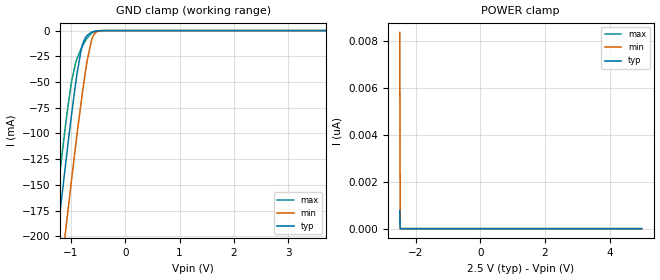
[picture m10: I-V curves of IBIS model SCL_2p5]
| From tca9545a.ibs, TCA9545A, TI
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|   Model
[Model]   SCL_2p5
Model_type   Input
Vinl = 0.75
Vinh = 1.75
|   typ   min   max
C_comp   3.453pF   3.557pF   3.722pF
[Voltage Range]   2.5   2.3   2.7
[Temperature Range]   27   125   -40
[Power Clamp Reference]   2.5   2.3   2.7
[GND Clamp Reference]   -0   -0   -0
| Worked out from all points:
|   GND clamp passes 1 mA (typ) near -0.59 V on its own axis
[GND Clamp]
|   Voltage   I(typ)   I(min)   I(max)
-2.5V     -804.8mA   -868.9mA   -764.9mA
-1.495V   -314.9mA   -380.7mA   -273.9mA
-1.24V    -194.1mA   -259.8mA   -153.7mA
-1.09V    -125.3mA   -190.2mA   -87.42mA
-985mV    -79.51mA   -142.7mA   -48.32mA
-917.5mV  -52.32mA   -113.1mA   -31.9mA
-812.5mV  -18.76mA   -69.19mA   -17.53mA
-700mV    -4.515mA   -28.64mA   -7.037mA
-625mV    -1.672mA   -10.1mA    -2.724mA
-550mV    -490.5uA   -2.124mA   -716.1uA
-407.5mV  -24.35uA   -73.49uA   -25.45uA
4.992V    0A         0A         0A
[POWER Clamp]
|   Voltage   I(typ)   I(min)   I(max)
-2.5V     761.4pA    8.365nA    500.7pA
-2.485V   0A         0A         0A
-2.478V   0A         0A         0A
4.992V    0A         0A         0A
